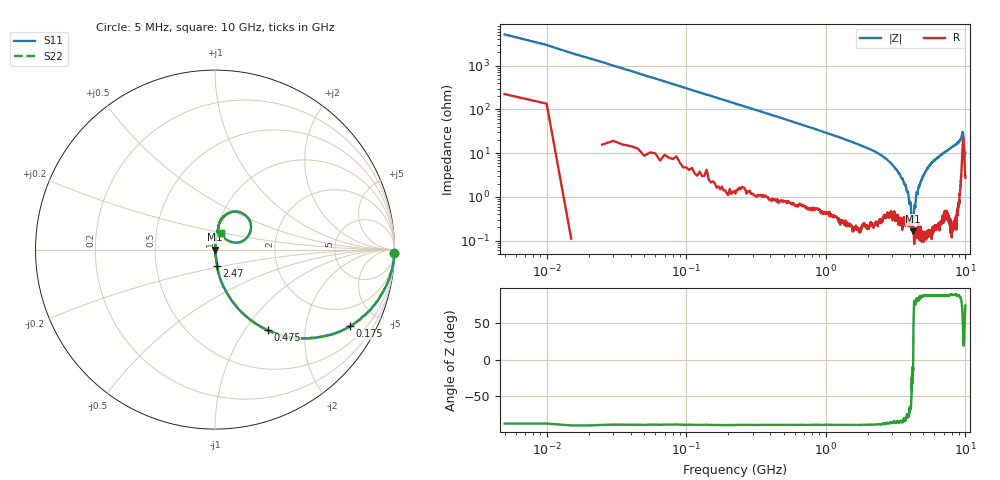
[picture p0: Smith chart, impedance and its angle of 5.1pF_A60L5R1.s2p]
! Amotech Co.,Ltd.
! http://www.amotech.co.kr/
! Part Number: A60L5R1
! These Parameters are Measured in Series Mode Connection
! Operation Temp=25[degC], DC Bias Voltage=0[V]
! Freq. Start=5[MHz] Stop=10[GHz], 2000[Steps]
! Date: Monday, July 14, 2020, 09:32:03
# GHZ S RI R 50.000000
!Freq.(Hz) S11(Real) S11(Imag) S21(Real) S21(Imag) S12(Real) S12(Imag) S22(Real) S22(Imag)
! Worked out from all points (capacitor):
!   2000 points, 5 MHz to 10 GHz, reference 50 ohm
!   read as one part in series: C = 5.24 pF near 55 MHz
!   lowest |Z| = 163 mohm at 4.23 GHz (marker M1)
!   series resonance near 4.225 GHz, so ESL is about 270 pH
!   S11 on the Smith chart (normalised r, x): 5 MHz: open; 175 MHz: 1.03, -3.51; 475 MHz: 1.02, -1.28; 2.47 GHz: 1.01, -0.18; 10 GHz: 1.05, +0.20
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0.005  0.9988 -0.0194  0.00122 0.0194  0.00122 0.0194  0.9988 -0.0194
0.08  0.931 -0.244  0.069 0.244  0.069 0.244  0.931 -0.244
0.175  0.7526 -0.4273  0.2474 0.4273  0.2474 0.4273  0.7526 -0.4273
0.475  0.2938 -0.4494  0.7062 0.4494  0.7062 0.4494  0.2938 -0.4494
0.89  0.1038 -0.2972  0.8962 0.2972  0.8962 0.2972  0.1038 -0.2972
1.675  0.0276 -0.1578  0.9724 0.1578  0.9724 0.1578  0.0276 -0.1578
2.47  0.0109 -0.0898  0.9891 0.0898  0.9891 0.0898  0.0109 -0.0898
3.34  0.00377 -0.034  0.9962 0.034  0.9962 0.034  0.00377 -0.034
3.88  0.00294 -0.0121  0.9971 0.0121  0.9971 0.0121  0.00294 -0.0121
4.05  0.0027 -0.00629  0.9973 0.00629  0.9973 0.00629  0.0027 -0.00629
4.165  0.00207 -0.00066  0.9979 0.00066  0.9979 0.00066  0.00207 -0.00066
4.23  0.00163 5.02e-05  0.9984 -5.02e-05  0.9984 -5.02e-05  0.00163 5.02e-05
4.31  0.00102 0.00605  0.999 -0.00605  0.999 -0.00605  0.00102 0.00605
4.465  0.00158 0.0119  0.9984 -0.0119  0.9984 -0.0119  0.00158 0.0119
5.005  0.00206 0.0306  0.9979 -0.0306  0.9979 -0.0306  0.00206 0.0306
5.725  0.00478 0.0594  0.9952 -0.0594  0.9952 -0.0594  0.00478 0.0594
6.67  0.0107 0.0891  0.9893 -0.0891  0.9893 -0.0891  0.0107 0.0891
8.335  0.0238 0.1454  0.9762 -0.1454  0.9762 -0.1454  0.0238 0.1454
9.55  0.1738 0.1873  0.8262 -0.1873  0.8262 -0.1873  0.1738 0.1873
9.64  0.1966 0.0993  0.8034 -0.0993  0.8034 -0.0993  0.1966 0.0993
9.83  0.0673 0.0531  0.9327 -0.0531  0.9327 -0.0531  0.0673 0.0531
10  0.0356 0.0928  0.9644 -0.0928  0.9644 -0.0928  0.0356 0.0928
